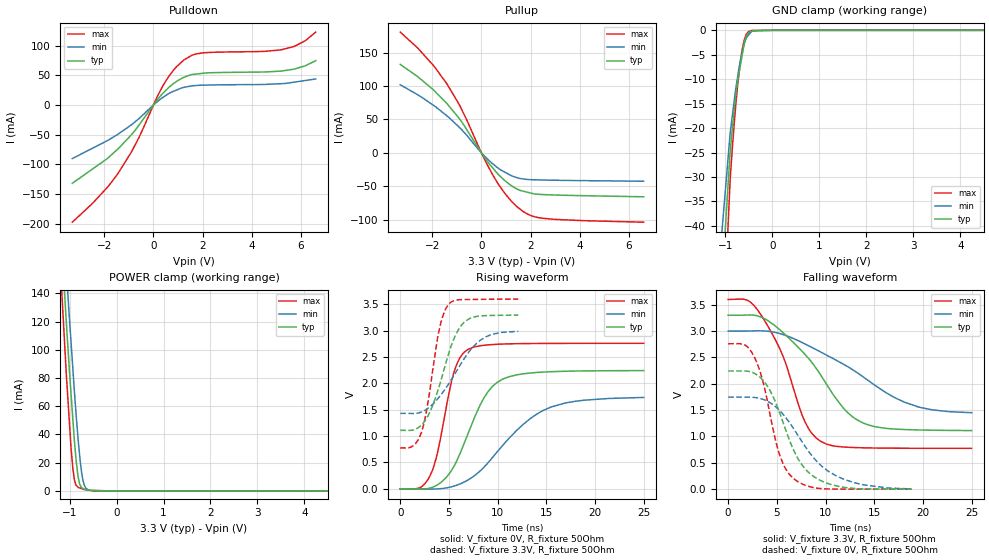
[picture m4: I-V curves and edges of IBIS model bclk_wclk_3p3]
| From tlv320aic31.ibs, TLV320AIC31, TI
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|   bclk_wclk_3p3 Model
[Model]   bclk_wclk_3p3
Model_type   I/O
Polarity   Non-Inverting
Enable   Active-Low
Vinl = 0.99
Vinh = 2.31
Vmeas = 1.65
Vref = 1.65
Cref = 10pF
Rref = 50
|   typ   min   max
|   (nom PVT)   (fast PVT)   (slow PVT)
|C_comp from frequency sweep method (F=25MHz)
|C_comp   1.371e-11   1.346e-11   1.385e-11
|ON state : BUFFER OUTPUT TURNED HIGH
|C_comp   1.914e-11   1.896e-11   1.958e-11
|OFF state: BUFFER IN HIGH IMPEDANCE
|C_comp   8.123e-12   7.961e-12   8.276e-12
|C_comp from LC tank measurement(L=1nH)
|Average
|Resonant Frequency(Hz)   2.085e+09   2.100e+09   2.075e+09
C_comp   5.886e-12   5.806e-12   5.944e-12
|ON state : BUFFER OUTPUT TURNED HIGH
|Resonant Frequency(Hz)   1.970e+09   1.980e+09   1.960e+09
|C_comp   6.533e-12   6.468e-12   6.600e-12
|OFF state: BUFFER IN HIGH IMPEDANCE
|Resonant Frequency(Hz)   2.200e+09   2.220e+09   2.190e+09
|C_comp   5.239e-12   5.145e-12   5.287e-12
| Where nom  PVT is Nominal Process, 3.3V, 26C
|   Fast PVT is Strong Process,  3.6V, -40C
|   Slow PVT is Weak Process,   3V, 86C
[Model Spec]
|Subparameter   typ   min   max
Vinl   0.99   0.9   1.08
Vinh   2.31   2.1   2.52
[Voltage Range]   3.3   3   3.6
|Ambient Temperature   25   85   -40
|Junction Temperature
[Temperature Range]   26   86   -40
[Pullup Reference]   3.3   3   3.6
[Pulldown Reference]   0   0   0
[Power Clamp Reference]   3.3   3   3.6
[GND Clamp Reference]   0   0   0
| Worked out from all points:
|   slope of the pulldown table from 0 to 0.495 V, typ, clamps not added: 20.5 ohm
|   slope of the pullup table from 0 to 0.495 V, typ, clamps not added: 20.4 ohm
|   GND clamp passes 1 mA (typ) near -0.54 V on its own axis
|   POWER clamp passes 1 mA (typ) near -0.66 V on its own axis
|   falling waveform, V_fixture 3.3V, R_fixture 50Ohm: 20-80 % time 5.53ns typ, 8.28ns min, 3.49ns max; typ from 3.3 V to 1.11 V
|   rising waveform, V_fixture 0V, R_fixture 50Ohm: 20-80 % time 3.26ns typ, 5.53ns min, 1.87ns max; typ from 0 V to 2.24 V
|   rising waveform, V_fixture 3.3V, R_fixture 50Ohm: 20-80 % time 2.29ns typ, 3.4ns min, 1.48ns max; typ from 1.11 V to 3.29 V
|   falling waveform, V_fixture 0V, R_fixture 50Ohm: 20-80 % time 3.11ns typ, 4.45ns min, 2.17ns max; typ from 2.24 V to 0.002 V
[Pulldown]
|   Voltage   I(typ)   I(min)   I(max)
-3.3V     -131.8mA   -90.22mA   -197.3mA
-2.48V    -107.8mA   -72.84mA   -165.7mA
-1.454V   -74.33mA   -49.41mA   -116.1mA
-896.4mV  -50.17mA   -33.4mA    -79.13mA
-583.2mV  -33.5mA    -22.75mA   -54.21mA
388.8mV   19.75mA    12.89mA    32.63mA
799.2mV   35.51mA    22.78mA    57.8mA
1.235V    46.42mA    29.66mA    75.62mA
1.962V    53.07mA    33.29mA    87.46mA
5.188V    56.96mA    35.83mA    92.69mA
6.178V    65.99mA    41.15mA    108.1mA
6.6V      74.56mA    43.72mA    122.6mA
[GND Clamp]
|   Voltage   I(typ)   I(min)   I(max)
-3.3V     -1.23A     -1.032A    -1.497A
-1.458V   -110.9mA   -85.23mA   -148mA
-897.6mV  -24.62mA   -20.95mA   -30.46mA
-842.4mV  -19.14mA   -16.7mA    -22.82mA
-792mV    -14.45mA   -12.85mA   -16.73mA
-745.8mV  -10.74mA   -9.904mA   -11.91mA
-691.2mV  -7.744mA   -6.739mA   -7.16mA
-601.2mV  -2.81mA    -2.923mA   -2.053mA
-554.4mV  -1.247mA   -1.567mA   -781.9uA
-500.4mV  -517.1uA   -904.9uA   -190.3uA
-285mV    -112.3uA   -3.923uA   -14uA
6.6V      0A         0A         0A
[Pullup]
|   Voltage   I(typ)   I(min)   I(max)
-3.3V     132.2mA    101.9mA    180.7mA
-2.592V   114mA      86.8mA     156.9mA
-1.958V   94.4mA     71.23mA    131mA
-1.393V   73.34mA    55.02mA    102.6mA
-896.4mV  51.11mA    38.16mA    71.84mA
54mV      -2.892mA   -2.188mA   -4.233mA
446.4mV   -22.1mA    -16.03mA   -32.15mA
950.4mV   -41.61mA   -29.04mA   -60.68mA
1.465V    -54.62mA   -37.56mA   -81.36mA
2.012V    -60.41mA   -40.28mA   -94.05mA
2.473V    -62.53mA   -40.81mA   -98.03mA
6.6V      -65.96mA   -42.71mA   -104mA
[POWER Clamp]
|   Voltage   I(typ)   I(min)   I(max)
-3.3V     1.472A     1.444A     1.575A
-1.162V   170.7mA    205.6mA    138.7mA
-1.073V   122mA      158.8mA    84.93mA
-1.017V   92.53mA    129.3mA    55.79mA
-968.4mV  69.04mA    105.5mA    30.57mA
-928.8mV  50.36mA    86.12mA    15.57mA
-896.4mV  35.2mA     70.26mA    7.799mA
-858mV    20.9mA     53.11mA    4.003mA
-810mV    8.775mA    33.75mA    2.431mA
-717mV    1.802mA    7.917mA    1.335mA
-591mV    579.9uA    556.2uA    478.2uA
6.6V      0A         0A         0A
[Ramp]
R_load = 50
|   typ   min   max
dV/dt_r   1.34441/3.24836e-09   1.03898/5.51311e-09   1.65495/1.86596e-09
dV/dt_f   1.31245/5.52881e-09   0.929281/8.27787e-09   1.69486/3.48169e-09
[Falling Waveform]
V_fixture = 3.3V
V_fixture_min = 3V
V_fixture_max = 3.6V
R_fixture = 50Ohm
|   Time   V(typ)   V(min)   V(max)
0s        3.3V       3V         3.6V
1.985ns   3.305V     3V         3.585V
3.445ns   3.26V      3.004V     3.286V
5.58ns    2.979V     2.938V     2.546V
7.905ns   2.554V     2.755V     1.273V
9.52ns    2.161V     2.601V     907mV
11.89ns   1.528V     2.366V     800.3mV
14.35ns   1.222V     2.067V     783.8mV
19.47ns   1.124V     1.564V     776.5mV
25ns      1.113V     1.451V     775.2mV
[Rising Waveform]
V_fixture = 0V
V_fixture_min = 0V
V_fixture_max = 0V
R_fixture = 50Ohm
|   Time   V(typ)   V(min)   V(max)
0s        1.04nV     4.553nV    682.2pV
1.97ns    -6.525mV   -2.019mV   14.7mV
3.08ns    14.79mV    -5.486mV   255.6mV
3.855ns   78.3mV     -2.068mV   705.9mV
5.505ns   421.5mV    49.4mV     2.202V
6.975ns   1.053V     168.1mV    2.643V
9.01ns    1.84V      491.4mV    2.728V
11.12ns   2.122V     947.2mV    2.748V
15.51ns   2.22V      1.551V     2.756V
25ns      2.241V     1.732V     2.758V
[Rising Waveform]
V_fixture = 3.3V
V_fixture_min = 3V
V_fixture_max = 3.6V
R_fixture = 50Ohm
|   Time   V(typ)   V(min)   V(max)
0s        1.109V     1.43V      774.3mV
1.335ns   1.115V     1.427V     816.6mV
2.18ns    1.208V     1.455V     1.072V
2.745ns   1.347V     1.512V     1.526V
3.925ns   1.898V     1.722V     2.943V
4.915ns   2.526V     1.973V     3.484V
5.905ns   2.995V     2.268V     3.582V
7.075ns   3.224V     2.6V       3.589V
9.27ns    3.286V     2.918V     3.594V
12.12ns   3.293V     2.985V     3.597V
[Falling Waveform]
V_fixture = 0V
V_fixture_min = 0V
V_fixture_max = 0V
R_fixture = 50Ohm
|   Time   V(typ)   V(min)   V(max)
0s        2.243V     1.747V     2.759V
1.68ns    2.243V     1.747V     2.741V
2.675ns   2.2V       1.742V     2.512V
3.565ns   2.069V     1.705V     2.047V
5.28ns    1.455V     1.494V     654mV
6.75ns    730mV      1.142V     197.5mV
8.45ns    287.7mV    670.6mV    44.04mV
11.14ns   61.4mV     249.6mV    3.29mV
13.96ns   6.087mV    81.64mV    1.752mV
18.86ns   1.769mV    5.191mV    967.1uV
